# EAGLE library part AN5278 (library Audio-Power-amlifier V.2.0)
The AN5278 is a monolithic integrated circuit designed for 4.8 W ´ 1 channel OTL (18 V, 8 W) output audio power amplifier suitable for TV application.
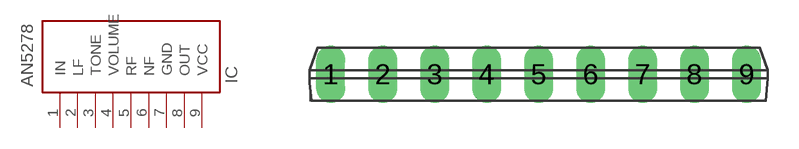
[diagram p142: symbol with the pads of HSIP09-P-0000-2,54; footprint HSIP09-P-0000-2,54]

Designator prefix IC

## AN5278  [HSIP09-P-0000-2,54]
1  IN  in
2  LF  in
3  TONE  in
4  VOLUME  in
5  RF  in
6  NF
7  GND  pwr
8  OUT  out
9  VCC  pwr

## Footprint HSIP09-P-0000-2,54 (pad centres in mm)
drill 0.9 long: 1 -10.16,0; 2 -7.62,0; 3 -5.08,0; 4 -2.54,0; 5 0,0; 6 2.54,0; 7 5.08,0; 8 7.62,0; 9 10.16,0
